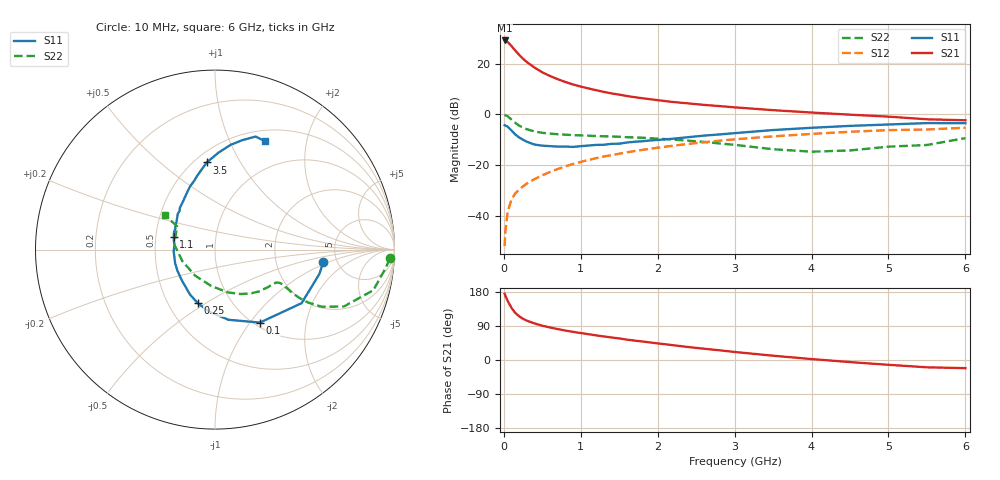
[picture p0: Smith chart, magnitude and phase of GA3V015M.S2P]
! Infineon Technologies  Discrete & RF Semiconductors
! BF775
! Si NPN RF Bipolar Junction Transistor in SOT23
! VCE = 3 V  IC = 15 mA
! Common Emitter S-Parameters:  May  1996
# GHz  S  MA  R  50
!  f  S11  S21  S12  S22
! GHz  MAG  ANG  MAG  ANG  MAG  ANG  MAG  ANG
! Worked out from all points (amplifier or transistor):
!   36 points, 10 MHz to 6 GHz, reference 50 ohm
!   highest |S21| = 29.1 dB at 10 MHz (marker M1)
!   |S21| within 3 dB of that: start of sweep to 121.9 MHz
!   unconditionally stable (mu >= 1): 448.7 MHz to 3.224 GHz
!   at 250 MHz: K = 0.80, MSG = 25.2 dB, |S12| = -28.4 dB
!   at 1.4 GHz: K = 1.11, MAG = 10.1 dB, |S12| = -16.1 dB
!   at 6 GHz: K = 0.96, MSG = 1.5 dB, |S12| = -5.3 dB
!   S11 on the Smith chart (normalised r, x): 10 MHz: 3.89, -0.86; 100 MHz: 1.06, -1.12; 250 MHz: 0.70, -0.46; 1.1 GHz: 0.62, +0.10; 3.5 GHz: 0.57, +0.73; 6 GHz: 0.63, +1.37
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0.01  0.607 -6.6  28.52 174.8  0.0025 88.3  0.9751 -2.9
0.02  0.5976 -13.0  28.14 169.6  0.0049 86.6  0.9577 -6.0
0.05  0.5675 -31.7  26.64 155.8  0.012 75.4  0.9107 -14.4
0.1  0.4774 -58.4  22.12 137.4  0.0209 68.6  0.7852 -23.8
0.15  0.398 -79.2  17.96 123.9  0.0277 65.3  0.6742 -28.2
0.2  0.3472 -95.4  14.81 115.2  0.0329 64.5  0.596 -29.6
0.25  0.3136 -107.8  12.41 108.6  0.0379 64.0  0.5413 -29.8
0.3  0.2866 -119.0  10.67 103.7  0.043 65.3  0.5049 -29.5
0.4  0.2523 -137.0  8.294 96.5  0.0525 66.6  0.4578 -28.3
0.5  0.2401 -150.7  6.716 90.5  0.0624 67.5  0.4298 -27.4
0.6  0.2348 -161.0  5.678 85.8  0.0728 67.5  0.4148 -27.2
0.7  0.2302 -169.5  4.922 81.5  0.0829 67.9  0.4037 -27.4
0.8  0.2306 -178.2  4.323 77.8  0.0938 67.5  0.395 -27.7
0.9  0.2268 173.7  3.864 74.3  0.1045 67.3  0.3878 -28.3
1.1  0.2414 162.6  3.226 68.1  0.1252 66.3  0.3771 -30.6
1.3  0.2501 152.1  2.756 62.2  0.1465 64.6  0.3677 -33.1
1.6  0.2771 139.4  2.29 53.8  0.1774 61.7  0.3528 -38.0
2.2  0.3292 121.7  1.743 39.0  0.2393 55.3  0.317 -50.1
3.5  0.488 95.4  1.204 11.3  0.3659 38.7  0.2041 -95.8
4.5  0.5895 81.6  0.981 -5.5  0.4511 25.3  0.1931 -160.7
5.5  0.6695 70.2  0.795 -19.3  0.4994 10.6  0.2474 148.5
6  0.6647 65.1  0.76 -21.5  0.5428 6.4  0.338 145.5
